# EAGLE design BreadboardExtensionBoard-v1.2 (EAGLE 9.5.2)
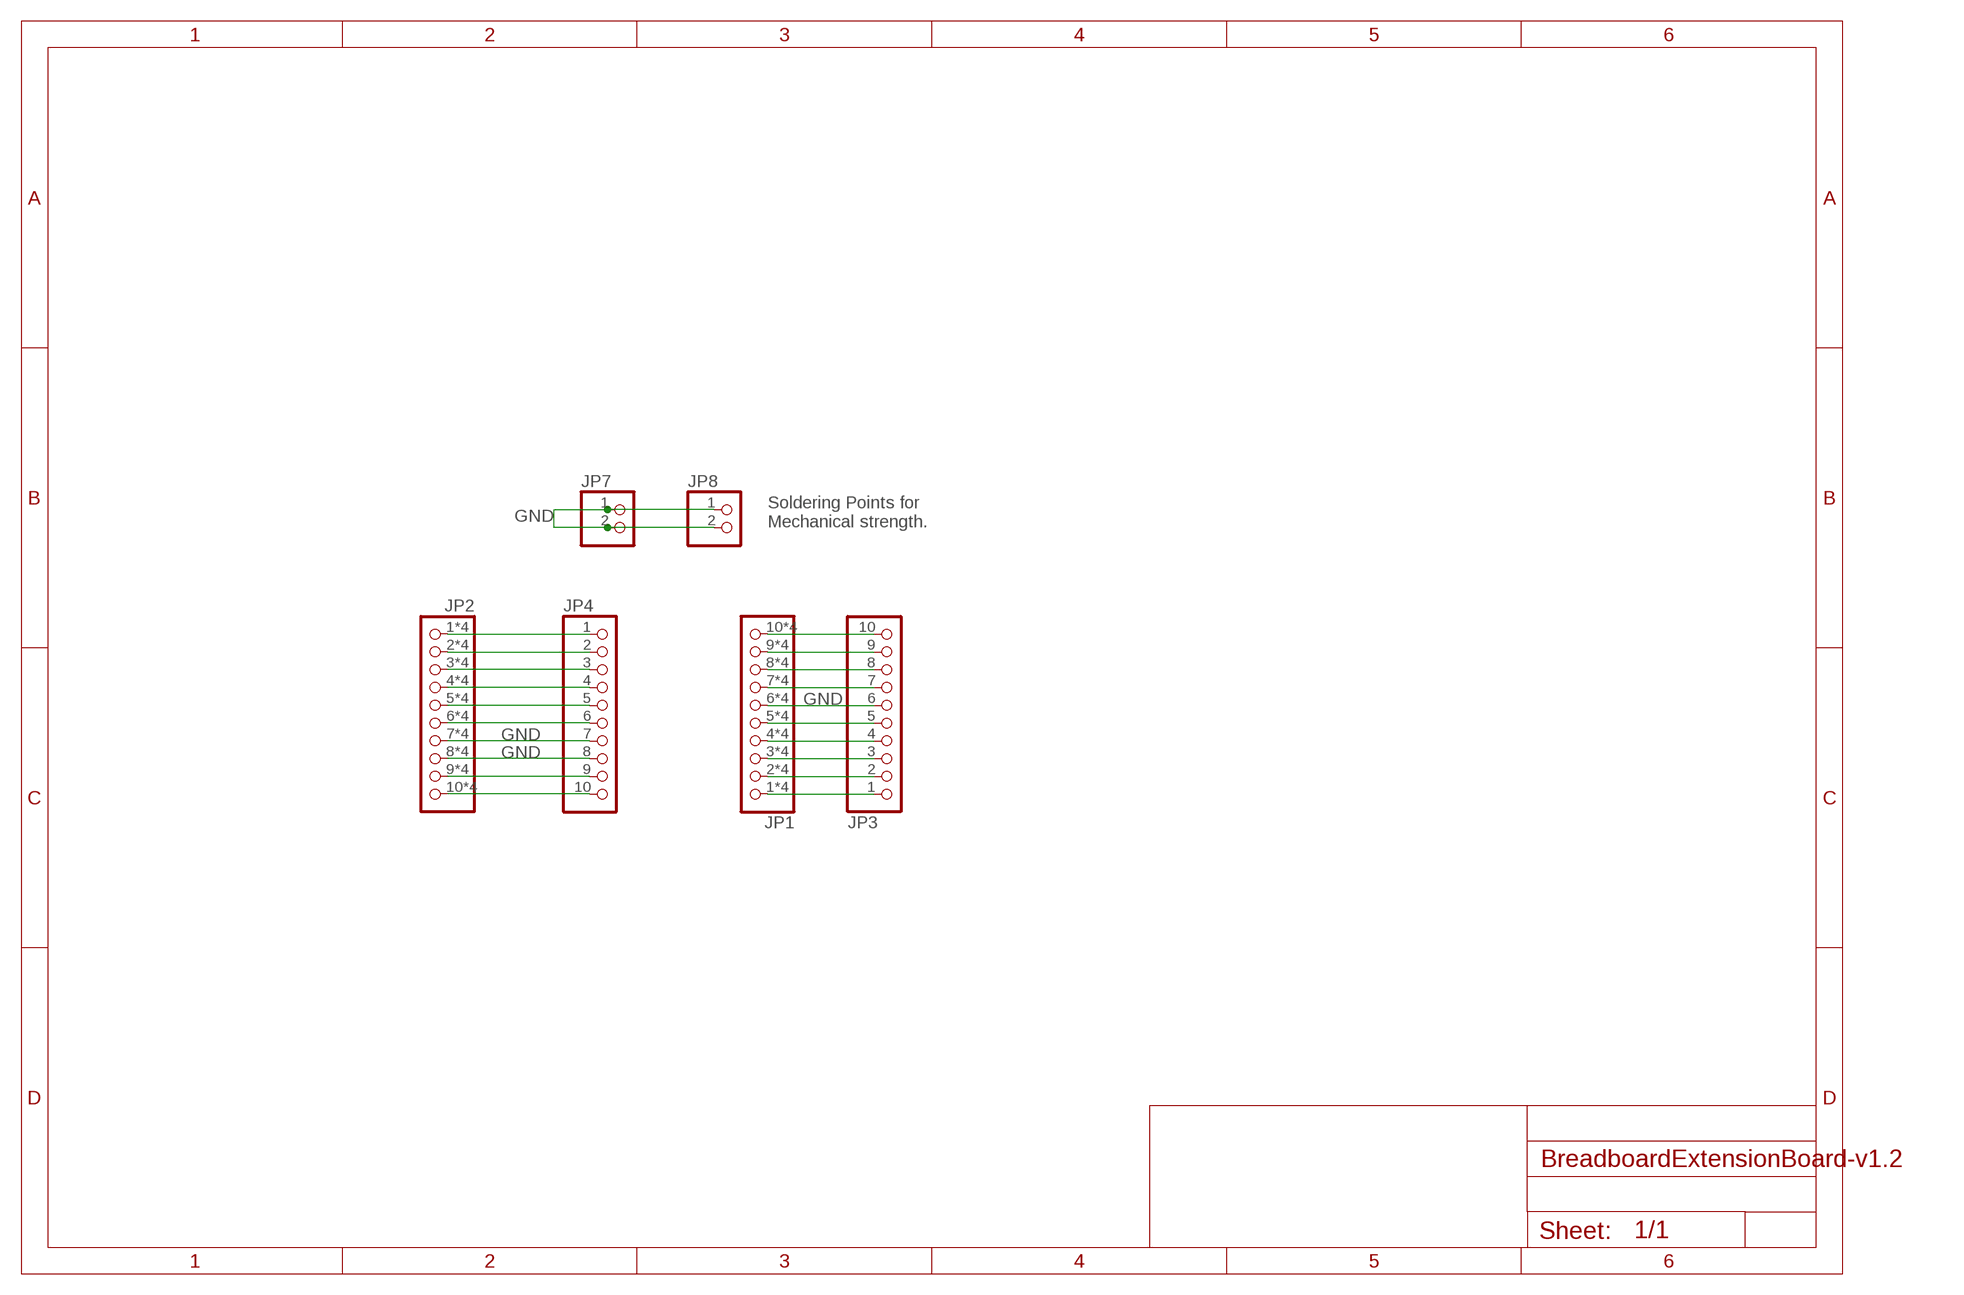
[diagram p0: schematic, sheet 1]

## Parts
JP1  PINHD-1X10_CATELLATED  [1X10TH/CASTELLATED]
JP2  PINHD-1X10_CATELLATED  [1X10TH/CASTELLATED]
JP3  PINHD-1X10  [1X10]
JP4  PINHD-1X10  [1X10]
JP7  PINHD-1X2_EXT  [1X02TH/EXT]
JP8  PINHD-1X2_EXT  [1X02TH/EXT]

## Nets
GND: JP1.6 JP1.B6 JP1.P$6 JP1.T6 JP2.7 JP2.8 JP2.B7 JP2.B8 JP2.P$7 JP2.P$8 JP2.T7 JP2.T8 JP3.6 JP4.7 JP4.8 JP7.1 JP7.2 JP8.1 JP8.2
N$1: JP2.1 JP2.B1 JP2.P$1 JP2.T1 JP4.1
N$2: JP2.2 JP2.B2 JP2.P$2 JP2.T2 JP4.2
N$3: JP1.3 JP1.B3 JP1.P$3 JP1.T3 JP3.3
N$4: JP1.4 JP1.B4 JP1.P$4 JP1.T4 JP3.4
N$5: JP1.5 JP1.B5 JP1.P$5 JP1.T5 JP3.5
N$7: JP1.7 JP1.B7 JP1.P$7 JP1.T7 JP3.7
N$8: JP1.8 JP1.B8 JP1.P$8 JP1.T8 JP3.8
N$9: JP1.9 JP1.B9 JP1.P$9 JP1.T9 JP3.9
N$10: JP1.10 JP1.B10 JP1.P$10 JP1.T10 JP3.10
N$11: JP1.2 JP1.B2 JP1.P$2 JP1.T2 JP3.2
N$12: JP1.1 JP1.B1 JP1.P$1 JP1.T1 JP3.1
N$13: JP2.3 JP2.B3 JP2.P$3 JP2.T3 JP4.3
N$14: JP2.4 JP2.B4 JP2.P$4 JP2.T4 JP4.4
N$15: JP2.5 JP2.B5 JP2.P$5 JP2.T5 JP4.5
N$16: JP2.6 JP2.B6 JP2.P$6 JP2.T6 JP4.6
N$19: JP2.9 JP2.B9 JP2.P$9 JP2.T9 JP4.9
N$20: JP2.10 JP2.B10 JP2.P$10 JP2.T10 JP4.10

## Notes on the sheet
- Soldering Points for 
  Mechanical strength.

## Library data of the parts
JP1 = WiPhone:PINHD-1X10: PIN HEADER
JP2-JP4 = MZJ:PINHD-1X10: PIN HEADER
JP7 JP8 = WiPhone:PINHD-1X2: PIN HEADER

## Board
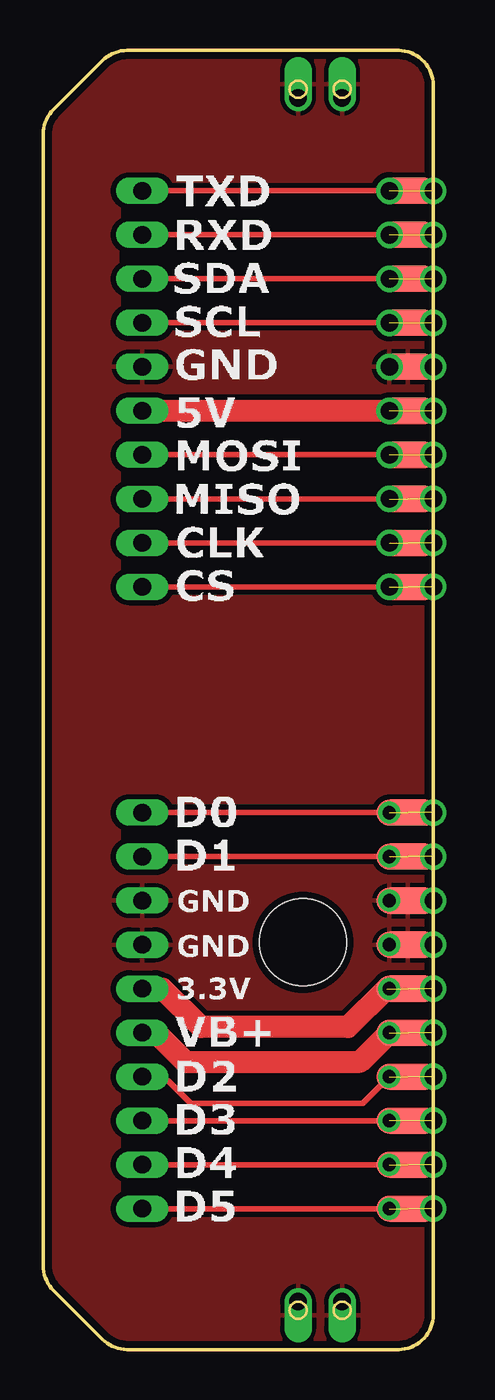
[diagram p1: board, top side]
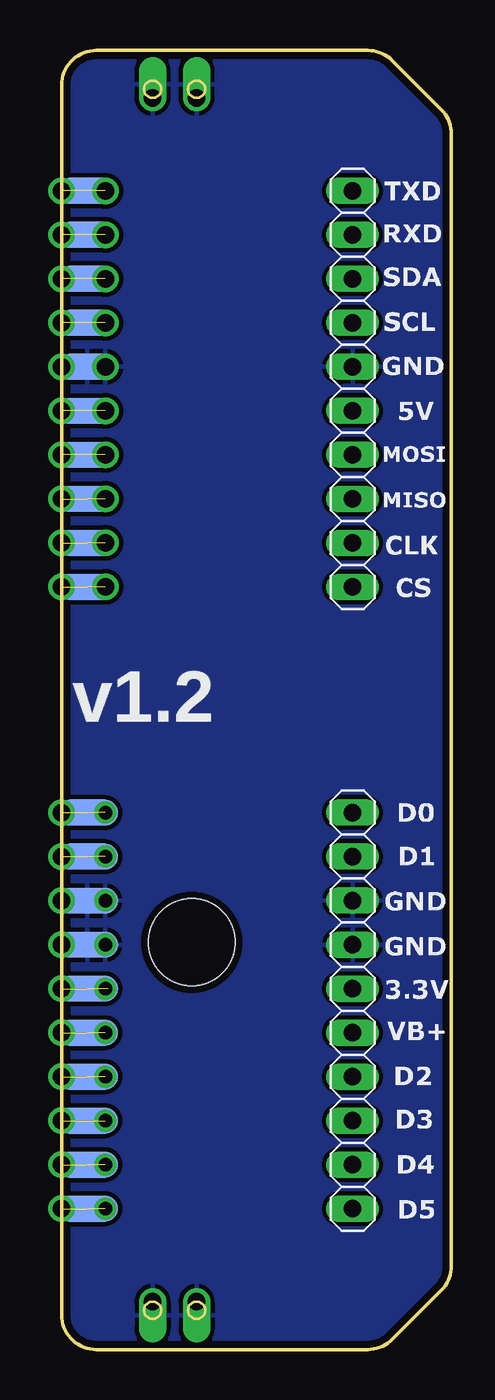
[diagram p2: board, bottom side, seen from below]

Size 22.5 x 75 mm. Coordinates in mm from the lower left corner, seen from the top.
Outline: 0,4.83 arc45 0.58,3.42 3.41,0.59 arc45 4.83,0 20.5,0 arc90 22.5,2 22.5,73 arc90 20.5,75 4.83,75 arc45 3.41,74.42 0.58,71.59 arc45 0,70.18 0,4.83
Copper layers (1*16): Top 0.035mm / dielectric 1.5mm / Bottom 0.035mm
Design rules "2LDaughterBoards": minimum track width 6mil, minimum drill 6mil, track to track 8mil, track to pad 8mil, pad to pad 8mil, via to via 8mil, smd to smd 0mil, copper to edge 16mil, drill to drill 6mil, minimum pad ring 10mil, minimum via ring 8mil, stop-mask expansion 4mil, vias tented up to drill 25mil, thermal gap 10mil
Holes 5 mm at 14.99,23.51
tRestrict: area 4.8,65.3 to 5.1,66; area 4.7,62.8 to 5,63.5; area 4.8,60.2 to 5.1,60.9; area 4.8,52.6 to 5.1,53.3; area 4.8,50.1 to 5.1,50.8; area 4.7,47.5 to 5,48.2; area 4.8,45 to 5.1,45.7; area 4.8,29.4 to 5.1,30.1; area 4.8,19.3 to 5.1,20; area 4.8,16.7 to 5.1,17.4; area 4.8,14.2 to 5.1,14.9; area 4.8,11.6 to 5.1,12.3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
bRestrict: area 13,21.5 to 17,25.5

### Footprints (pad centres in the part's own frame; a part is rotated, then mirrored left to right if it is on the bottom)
1X10TH/CASTELLATED = drill 1 pad 1.5: 1 2.54,-11.43; 2 2.54,-8.89; 3 2.54,-6.35; 4 2.54,-3.81; 5 2.54,-1.27; 6 2.54,1.27; 7 2.54,3.81; 8 2.54,6.35; 9 2.54,8.89; 10 2.54,11.43 | smd 3.565 x 1.5 bottom: B1 1.055,-11.43; B2 1.055,-8.89; B3 1.055,-6.35; B4 1.055,-3.81; B5 1.055,-1.27; B6 1.055,1.27; B7 1.055,3.81; B8 1.055,6.35; B9 1.055,8.89; B10 1.055,11.43 | drill 1.016: P$1 0,-11.43; P$2 0,-8.89; P$3 0,-6.35; P$4 0,-3.81; P$5 0,-1.27; P$6 0,1.27; P$7 0,3.81; P$8 0,6.35; P$9 0,8.89; P$10 0,11.43 | smd 3.565 x 1.5: T1 1.055,-11.43; T2 1.055,-8.89; T3 1.055,-6.35; T4 1.055,-3.81; T5 1.055,-1.27; T6 1.055,1.27; T7 1.055,3.81; T8 1.055,6.35; T9 1.055,8.89; T10 1.055,11.43
1X10TH/CASTELLATED' = drill 1 pad 1.5: 1 2.54,-11.43; 2 2.54,-8.89; 3 2.54,-6.35; 4 2.54,-3.81; 5 2.54,-1.27; 6 2.54,1.27; 7 2.54,3.81; 8 2.54,6.35; 9 2.54,8.89; 10 2.54,11.43 | smd 3.565 x 1.5 bottom: B1 1.055,-11.43; B2 1.055,-8.89; B3 1.055,-6.35; B4 1.055,-3.81; B5 1.055,-1.27; B6 1.055,1.27; B7 1.055,3.81; B8 1.055,6.35; B9 1.055,8.89; B10 1.055,11.43 | drill 0.762: P$1 0,-11.43; P$2 0,-8.89; P$3 0,-6.35; P$4 0,-3.81; P$5 0,-1.27; P$6 0,1.27; P$7 0,3.81; P$8 0,6.35; P$9 0,8.89; P$10 0,11.43 | smd 3.565 x 1.5: T1 1.055,-11.43; T2 1.055,-8.89; T3 1.055,-6.35; T4 1.055,-3.81; T5 1.055,-1.27; T6 1.055,1.27; T7 1.055,3.81; T8 1.055,6.35; T9 1.055,8.89; T10 1.055,11.43
1X10 = drill 1.016 long: 1 -11.43,0; 2 -8.89,0; 3 -6.35,0; 4 -3.81,0; 5 -1.27,0; 6 1.27,0; 7 3.81,0; 8 6.35,0; 9 8.89,0; 10 11.43,0
1X02TH/EXT = drill 1.016 pad 1.575 offset: 1 0,-2.54; 2 0,0

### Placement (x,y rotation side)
JP1  19.97,55.46 0 top
JP2  [1X10TH/CASTELLATED']  19.97,19.56 0 top
JP3  5.71,55.46 90 bottom
JP4  5.71,19.56 90 bottom
JP7  17.25,2.76 270 top
JP8  14.71,72.26 90 top

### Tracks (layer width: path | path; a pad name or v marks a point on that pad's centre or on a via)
GND
  pour Top (isolate 0.305): 0.01,70.29 0.01,4.69 arc90 4.71,-0.01 20.41,-0.01 arc90 22.51,2.09 22.51,72.89 arc90 20.41,74.99 4.71,74.99 arc90
  pour Bottom (isolate 0.254): -0.09,70.29 -0.09,4.69 arc90 4.61,-0.01 20.31,-0.01 arc90 22.41,2.09 22.41,72.89 arc90 20.31,74.99 4.61,74.99 arc90
N$1  (3 unrouted)
  Top 0.305: JP4.1 JP2.B1
N$2  (4 unrouted)
  Top 0.305: 20.1,10.67 JP4.2
N$3  (4 unrouted)
  Top 0.305: 20.1,49.11 JP3.3
N$4  (3 unrouted)
  Top 0.305: JP3.4 JP1.P$4
N$5  (3 unrouted)
  Top 1.27: JP3.5 JP1.P$5
N$7  (3 unrouted)
  Top 0.305: JP1.T7 JP3.7
N$8  (4 unrouted)
  Top 0.305: 20.2,61.81 JP3.8
N$9  (3 unrouted)
  Top 0.305: JP1.T9 JP3.9
N$10  (3 unrouted)
  Top 0.305: JP3.10 JP1.P$10
N$11  (4 unrouted)
  Top 0.305: 20,46.57 JP3.2
N$12  (3 unrouted)
  Top 0.305: JP1.B1 JP3.1
N$13  (3 unrouted)
  Top 0.305: JP4.3 JP2.B3
N$14  (3 unrouted)
  Top 0.305: JP4.4 5.95,15.51 7.2,15.51 8.5,14.21 18.43,14.21 JP2.P$4
N$15  (3 unrouted)
  Top 1.27: JP4.5 6.52,18.29 8.2,16.61 18.29,16.61 JP2.P$5
N$16  (4 unrouted)
  Top 1.27: JP4.6 6.88,20.83 9.1,18.61 17.6,18.61 19.82,20.83
N$19  (4 unrouted)
  Top 0.305: 20.1,28.45 JP4.9
N$20  (4 unrouted)
  Top 0.305: 20.2,30.99 JP4.10

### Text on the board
bPlace: v1.2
